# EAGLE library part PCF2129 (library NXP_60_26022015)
Accurate RTC with integrated quartz crystal for industrial The PCF2129T is a CMOS1 Real Time Clock (RTC) and calendar with an integrated Temperature Compensated Crystal (Xtal) Oscillator (TCXO) and a 32.768 kHz quartz crystal optimized for very high accuracy and very low power consumption. The PCF2129T has a selectable I2C-bus or SPI-bus, a backup battery switch-over circuit, a programmable watchdog function, a timestamp function, and many other features. AAL Eindhoven MK
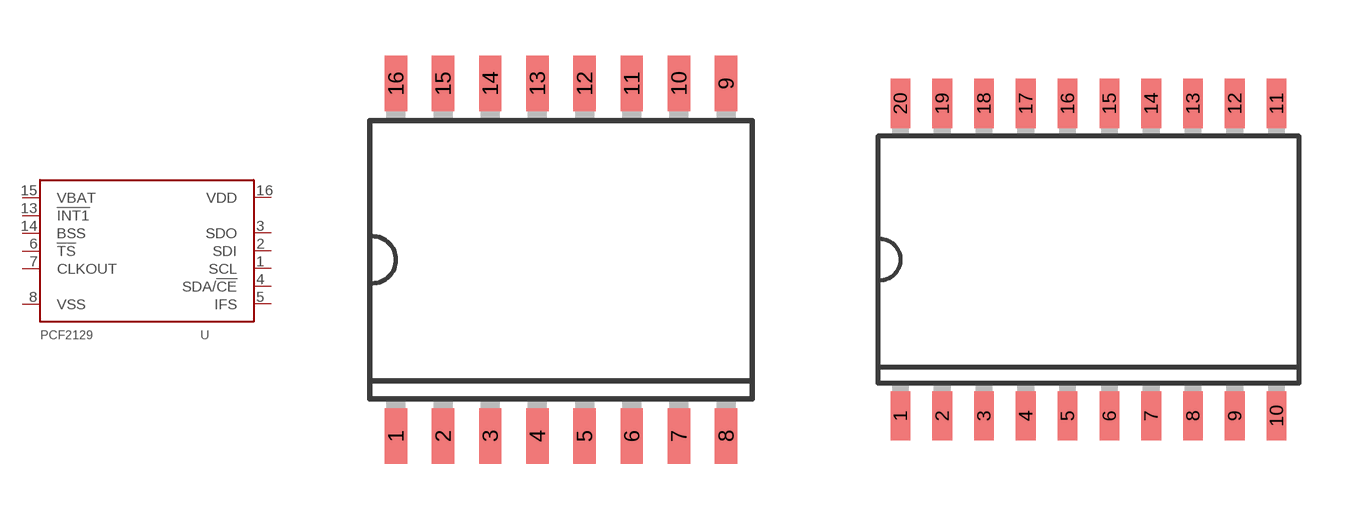
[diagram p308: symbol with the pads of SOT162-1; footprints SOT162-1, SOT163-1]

Designator prefix U

## PCF2129T (TEMPERATURE_RANGE: -15 °C to +60 °C)  [SOT162-1]
1  SCL
2  SDI  in
3  SDO  out
4  SDA/!CE  in
5  IFS  in
6  !TS!  in
7  CLKOUT  out
8  VSS  pwr
13  !INT1!  out
14  BSS  out
15  VBAT  pwr
16  VDD  pwr

## PCF2129AT (TEMPERATURE_RANGE: -15 °C to +60 °C)  [SOT163-1]
1  SCL
2  SDI  in
3  SDO  out
4  SDA/!CE  in
5  IFS  in
6  !TS!  in
7  CLKOUT  out
8  VSS  pwr
17  !INT1!  out
18  BSS  out
19  VBAT  pwr
20  VDD  pwr

## Footprint SOT162-1 (pad centres in mm)
SOT162-1 SO16: plastic small outline package; 16 leads; body width 7.5 mm JEDEC: -- IEC: --
smd 0.6 x 1.5: 1 -4.445,-4.75; 2 -3.175,-4.75; 3 -1.905,-4.75; 4 -0.635,-4.75; 5 0.635,-4.75; 6 1.905,-4.75; 7 3.175,-4.75; 8 4.445,-4.75; 9 4.445,4.75; 10 3.175,4.75; 11 1.905,4.75; 12 0.635,4.75; 13 -0.635,4.75; 14 -1.905,4.75; 15 -3.175,4.75; 16 -4.445,4.75

## Footprint SOT163-1 (pad centres in mm)
SOT163-1 SO20: plastic small outline package; 20 leads; body width 7.5 mm JEDEC: MS-013 IEC: 075E04
smd 0.6 x 1.5: 1 -5.715,-4.75; 2 -4.445,-4.75; 3 -3.175,-4.75; 4 -1.905,-4.75; 5 -0.635,-4.75; 6 0.635,-4.75; 7 1.905,-4.75; 8 3.175,-4.75; 9 4.445,-4.75; 10 5.715,-4.75; 11 5.715,4.75; 12 4.445,4.75; 13 3.175,4.75; 14 1.905,4.75; 15 0.635,4.75; 16 -0.635,4.75; 17 -1.905,4.75; 18 -3.175,4.75; 19 -4.445,4.75; 20 -5.715,4.75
